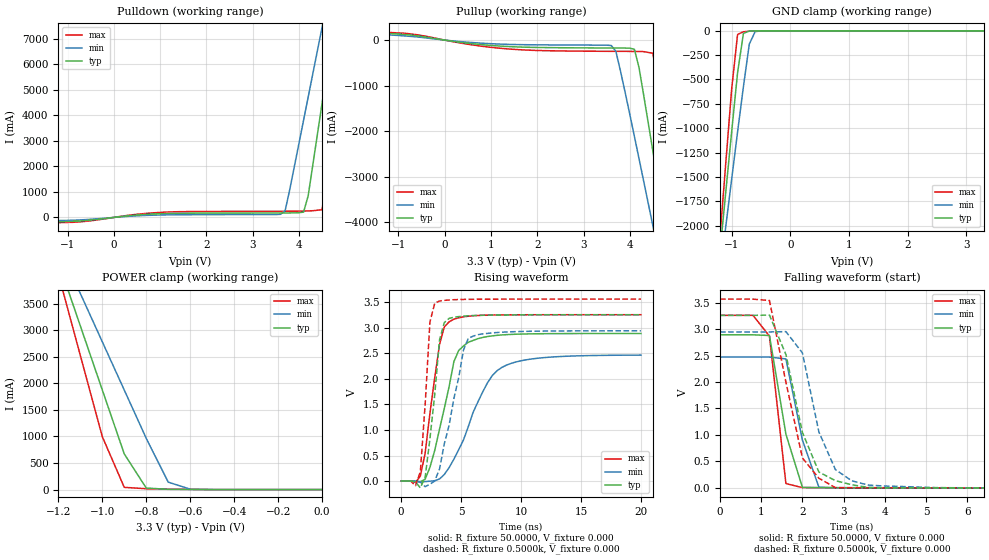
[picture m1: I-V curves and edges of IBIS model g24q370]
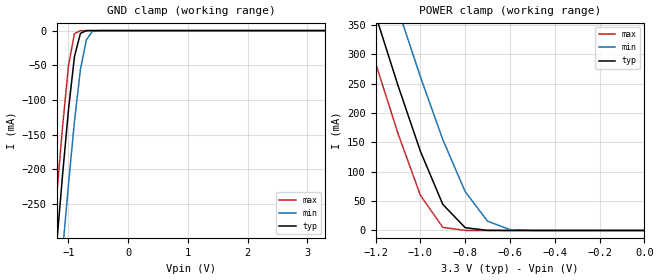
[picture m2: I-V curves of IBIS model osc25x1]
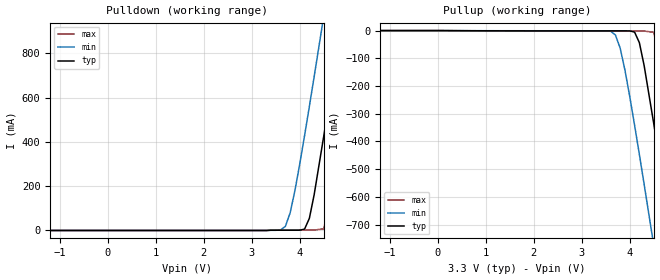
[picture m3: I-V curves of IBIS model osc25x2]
|   National Semiconductor Corporation
|   Interface Products Group
|   IBIS Model of DP83849
|   80L LQFP Package
[IBIS Ver]   4.2
[Comment char]  |_char
[File name]   dp83849.ibs
[File Rev]   1.1
[Date]   09/07/2010
[Source]   File originated at National Semiconductor Corporation.
   Interface Group/Analog Division. All models created with
   Spectre s2ibis simulations by Sida Zhang.
   Originally Created on 8/24/2005 by Sida Zhang, modified
   on 9/07/2010 by Peggy Alavi
[Notes]
   Rev 0.1 The pins TPTDP, TPTDM, TPRDP, and TPRDM are
   high-speed analog I/O pins. Models of these pins are
   not available due to the IBIS modeling limitations
   and design complexity.
   Rev 1.1 removes model selector. Model selector included a
   production test mode which is not available in the final
   product.
Begin IBIS Parser Results
| Do NOT edit this section manually!
Checking ...\dp83849.ibs for IBIS 4.2 Compatibility...
WARNING - Model osc25x1: POWER Clamp : Typical value never becomes zero
WARNING - Model osc25x1: POWER Clamp : Minimum value never becomes zero
WARNING - Model osc25x1: POWER Clamp : Maximum value never becomes zero
Errors  : 0
Warnings: 3
File Passed
| End IBIS Parser Results
[Disclaimer]
(C) Copyright National Semiconductor Corporation 2010
   All rights reserved
   National Semiconductor Corporation hereby grants
the user of this IBIS model a non-exclusive, nontransferable
license to use this IBIS model under the following terms.
Before using this IBIS model, the user should read this
license.  If the user does not accept these terms,  the
IBIS model should be returned to National within 30 days.
   The user is granted this license only to use the
IBIS model and is not granted rights to sell, load, rent,
lease or license the IBIS model in whole or in part, or in
modified form to anyone other than user. User may modify
the IBIS model to suit its specific applications but rights
to derivative works and such modifications shall belong to
National.
   This IBIS model is provided on an "AS IS" basis and
National makes absolutely no warranty with respect to the
information contained herein.NATIONAL DISCLAIMS AND CUSTOMER
WAIVES ALL WARRANTIES, EXPRESS OR IMPLIED, INCLUDING
WARRANTIES OF MERCHANTABILITY OR FITNESS FOR A PARTICULAR
PURPOSE. The entire risk as to quality and performance is
with the Customer. ACCORDINGLY, IN NO EVENT SHALL THE
COMPANY BE LIABLE FOR ANY DAMAGES, WHETHER IN CONTRACT OR
TORT,INCLUDING ANY LOST PROFITS OR OTHER INCIDENTAL,
CONSEQUENTIAL, EXEMPLARY, OR PUNITIVE DAMAGES ARISING OUT
OF THE USE OR APPLICATION OF THE IBIS model provided in
this package.Further, National reserves the right to make
changes without notice to any product herein to improve
reliability, function, or design. National does not convey
any license under patent rights or any other intellectual
property rights, including those of third parties.
   National is not obligated to provide maintenance or support
for the licensed IBIS model.
[Copyright]   Copyright 2010, National Semiconductor, All Rights Reserved
[Component]   DP83849
[Manufacturer]  National Semiconductor Corporation
[Package]
|   typ   min   max
R_pkg   0.171   0.153   0.189
L_pkg   5.515nH   4.604nH   6.091nH
C_pkg   0.126pF   0.090p   0.273p
[Pin]   signal_name   model_name   R_pin   L_pin   C_pin
1   CRS_A   g24q370   0.18332   5.99n   0.273p
2   RX_ER_A   g24q370   0.1772   5.642n   0.124p
3   COL_A   g24q370   0.17474   5.41n   0.105p
4   RXD0_A   g24q370   0.17112   5.202n   0.097p
5   RXD1_A   g24q370   0.16808   5.036n   0.092p
6   COREGND1   GND   0.1654   4.894n   0.09p
7   PFBIN1   NC   0.16363   4.792n   0.09p
8   RXD2_A   g24q370   0.16189   4.711n   0.093p
9   RXD3_A   g24q370   0.16103   4.653n   0.102p
10   IOGND1   GND   0.15937   4.604n   0.183p
11   IOVDD1   POWER   0.15311   4.633n   0.184p
12   TX_CLK_A   g24q370   0.16419   4.867n   0.103p
13   TX_EN_A   g24q370   0.17125   4.867n   0.095p
14   TXD0_A   g24q370   0.17056   4.854n   0.092p
15   TXD1_A   g24q370   0.17201   4.92n   0.094p
16   TXD2_A   g24q370   0.17334   4.989n   0.095p
17   TXD3_A   g24q370   0.17521   5.099n   0.1p
18   PWRDOWN_INT_A   g24q370   0.17779   5.236n   0.105p
19   LED_LINK_A   g24q370   0.18792   5.842n   0.124p
20   LED_SPEED_A   g24q370   0.1893   6.091n   0.271p
21   LED_ACT/COL_A   g24q370   0.18332   5.99n   0.273p
22   ANAGND1   GND   0.1772   5.642n   0.124p
23   TPRDM_A   NC   0.17474   5.41n   0.105p
24   TPRDP_A   NC   0.17112   5.202n   0.097p
25   CDGND1   GND   0.16808   5.036n   0.092p
26   TPTDM_A   NC   0.1654   4.894n   0.09p
27   TPTDP_A   NC   0.16363   4.792n   0.09p
28   PFBIN2   NC   0.16189   4.711n   0.093p
29   ANAGND2   GND   0.16103   4.653n   0.102p
30   ANA33VDD   POWER   0.15937   4.604n   0.183p
31   PFBOUT   NC   0.15311   4.633n   0.184p
32   RBIAS   NC   0.16419   4.867n   0.103p
33   ANAGND3   GND   0.17125   4.867n   0.095p
34   PFBIN3   NC   0.17056   4.854n   0.092p
35   TPTDP_B   NC   0.17201   4.92n   0.094p
36   TPTDM_B   NC   0.17334   4.989n   0.095p
37   CDGND2   GND   0.17521   5.099n   0.1p
38   TPRDP_B   NC   0.17779   5.236n   0.105p
39   TPRDM_B   NC   0.18792   5.842n   0.124p
40   ANAGND4   GND   0.1893   6.091n   0.271p
41   LED_ACT/COL_B   g24q370   0.18332   5.99n   0.273p
42   LED_SPEED_B   g24q370   0.1772   5.642n   0.124p
43   LED_LINK_B   g24q370   0.17474   5.41n   0.105p
44   PWRDOWN_INT_B   g24q370   0.17112   5.202n   0.097p
45   TXD3_B   g24q370   0.16808   5.036n   0.092p
46   TXD2_B   g24q370   0.1654   4.894n   0.09p
47   TXD1_B   g24q370   0.16363   4.792n   0.09p
48   TXD0_B   g24q370   0.16189   4.711n   0.093p
49   TX_EN_B   g24q370   0.16103   4.653n   0.102p
50   TX_CLK_B   g24q370   0.15937   4.604n   0.183p
51   IOVDD2   POWER   0.15311   4.633n   0.184p
52   IOGND2   GND   0.16419   4.867n   0.103p
53   RXD3_B   g24q370   0.17125   4.867n   0.095p
54   PFBIN4   NC   0.17056   4.854n   0.092p
55   COREGND2   GND   0.17201   4.92n   0.094p
56   RXD2_B   g24q370   0.17334   4.989n   0.095p
57   RXD1_B   g24q370   0.17521   5.099n   0.1p
58   RXD0_B   g24q370   0.17779   5.236n   0.105p
59   COL_B   g24q370   0.18792   5.842n   0.124p
60   RX_ER_B   g24q370   0.1893   6.091n   0.271p
61   CRS_B   g24q370   0.18332   5.99n   0.273p
62   RX_DV_B   g24q370   0.1772   5.642n   0.124p
63   RX_CLK_B   g24q370   0.17474   5.41n   0.105p
64   IOGND3   GND   0.17112   5.202n   0.097p
65   IOVDD3   POWER   0.16808   5.036n   0.092p
66   MDIO   g24q370   0.1654   4.894n   0.09p
67   MDC   g24q370   0.16363   4.792n   0.09p
68   CLK2MAC   g24q370   0.16189   4.711n   0.093p
69   X2   osc25x2   0.16103   4.653n   0.102p
70   X1   osc25x1   0.15937   4.604n   0.183p
71   RESET_N   g24q370   0.15311   4.633n   0.184p
72   TCK   g24q370   0.16419   4.867n   0.103p
73   TDO   g24q370   0.17125   4.867n   0.095p
74   TMS   g24q370   0.17056   4.854n   0.092p
75   TRST_N   g24q370   0.17201   4.92n   0.094p
76   TDI   g24q370   0.17334   4.989n   0.095p
77   IOGND4   GND   0.17521   5.099n   0.1p
78   IOVDD4   POWER   0.17779   5.236n   0.105p
79   RX_CLK_A   g24q370   0.18792   5.842n   0.124p
80   RX_DV_A   g24q370   0.1893   6.091n   0.271p
[Diff_pin]   inv_pin   vdiff   tdelay_typ   tdelay_min   tdelay_max
| The '+' pin is Diff_pin and the '-' pin is the inv_pin
24   23   0.100   0 0 0
27   26   0.100   0 0 0
35   36   0.100   0 0 0
38   39   0.100   0 0 0
| Models and submodels in the file (3): g24q370 (I/O), osc25x1 (Input), osc25x2 (Output)
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|   Model g24q370
[Model]   g24q370
Model_type   I/O
Polarity   Non-Inverting
Enable   Active-High
Vinl = 0.8000V
Vinh = 2.0000V
Vmeas = 1.5000V
C_comp   1.0640pF   1.0620pF   1.0670pF
[Temperature Range]   25.0000   0.1250k   -40.0000
[Voltage Range]   3.3000V   3.0000V   3.6000V
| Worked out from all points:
|   slope of the pulldown table from 0 to 0.495 V, typ, clamps not added: 5.31 ohm
|   slope of the pullup table from 0 to 0.495 V, typ, clamps not added: 7.25 ohm
|   GND clamp passes 1 mA (typ) near -0.64 V on its own axis
|   POWER clamp passes 1 mA (typ) near -0.54 V on its own axis
|   rising waveform, R_fixture 50.0000, V_fixture 0.000: 20-80 % time 1.6ns typ, 2.8ns min, 1.1ns max; typ from 0 V to 2.89 V
|   rising waveform, R_fixture 0.5000k, V_fixture 0.000: 20-80 % time 833ps typ, 1.56ns min, 573ps max; typ from 0 V to 3.26 V
|   falling waveform, R_fixture 50.0000, V_fixture 0.000: 20-80 % time 452ps typ, 464ps min, 281ps max; typ from 2.89 V to 0 V
|   falling waveform, R_fixture 0.5000k, V_fixture 0.000: 20-80 % time 659ps typ, 611ps min, 580ps max; typ from 3.26 V to 0 V
[Pulldown]
| voltage   I(typ)   I(min)   I(max)
-3.3V     -160.5mA   -118.3mA   -200.7mA
-900mV    -153.7mA   -111mA     -192.4mA
1.1V      151.8mA    98.11mA    206.2mA
3.6V      174.1mA    121.6mA    241.2mA
3.7V      174.7mA    254.1mA    242mA
4.1V      208.2mA    3.809A     248.7mA
4.2V      852.2mA    4.721A     254.3mA
4.5V      4.477A     7.457A     302mA
4.7V      6.898A     9.283A     2.796A
4.9V      9.321A     11.11A     5.87A
5.1V      11.75A     12.94A     8.947A
6.6V      30.05A     26.73A     32.17A
[Pullup]
| voltage   I(typ)   I(min)   I(max)
-3.3V     188.1mA    165.2mA    206.9mA
-900mV    123.6mA    93.95mA    153.1mA
1.3V      -138.1mA   -91.87mA   -188.7mA
3.6V      -174.3mA   -119.7mA   -247.2mA
3.7V      -174.6mA   -248.3mA   -247.7mA
4.1V      -202.3mA   -2.118A    -249.5mA
4.2V      -607mA     -2.608A    -250.6mA
4.5V      -2.447A    -4.087A    -288.9mA
4.7V      -3.699A    -5.076A    -1.602A
4.9V      -4.956A    -6.068A    -3.14A
5.1V      -6.215A    -7.061A    -4.687A
6.6V      -15.68A    -14.52A    -16.34A
[GND_clamp]
| voltage   I(typ)   I(min)   I(max)
-3.3V     -15.47A    -12.9A     -18.37A
-1.2V     -2.269A    -2.494A    -2.116A
-1.1V     -1.647A    -2.005A    -1.349A
-1V       -1.031A    -1.519A    -592.6mA
-900mV    -430.7mA   -1.039A    -37.49mA
-800mV    -26.32mA   -572.9mA   -9.444mA
-700mV    -1.926mA   -136.4mA   -3.598mA
-600mV    -247.7uA   -8.119mA   -648.8uA
-400mV    -1.571uA   -27.47uA   -1.62uA
3.3V      22.02pA    3.648uA    15.2pA
[POWER_clamp]
| voltage   I(typ)   I(min)   I(max)
-3.3V     29.64A     23.74A     36.19A
-1.2V     4.29A      4.604A     4.058A
-1.1V     3.083A     3.693A     2.528A
-1V       1.877A     2.784A     997.8mA
-900mV    671.8mA    1.874A     42.61mA
-800mV    29.37mA    964.9mA    16.3mA
-700mV    5.409mA    140.5mA    9.688mA
-600mV    1.864mA    8.479mA    4.466mA
0V        22.02pA    589.3pA    18.15pA
[Ramp]
| variable   typ   min   max
dV/dt_r   1.7348/1.6680n   1.4811/3.0471n   1.9560/1.1060n
dV/dt_f   1.8068/1.8411n   1.5594/3.2593n   2.0132/1.2189n
R_load = 50.0000
[Rising Waveform]
R_fixture = 50.0000
V_fixture = 0.000
V_fixture_min = 0.000
V_fixture_max = 0.000
| time   V(typ)   V(min)   V(max)
0s        121pV      6.465nV    36.64pV
1.6ns     -12.04mV   -15.26mV   96.9mV
2ns       34.22mV    -11.2mV    543.1mV
2.4ns     268mV      -3.569mV   1.326V
3.2ns     1.016V     39.7mV     2.674V
4ns       1.85V      262mV      3.12V
4.8ns     2.559V     613.5mV    3.2V
7.2ns     2.832V     1.925V     3.252V
8.4ns     2.864V     2.227V     3.257V
20ns      2.891V     2.468V     3.26V
[Rising Waveform]
R_fixture = 0.5000k
V_fixture = 0.000
V_fixture_min = 0.000
V_fixture_max = 0.000
| time   V(typ)   V(min)   V(max)
0s        130pV      7.171nV    38.79pV
1.2ns     -20.26mV   28.89uV    -92.41mV
1.6ns     -134.2mV   -21.16mV   180.7mV
2ns       72.06mV    -111.1mV   1.492V
2.4ns     825.8mV    -63.59mV   3.114V
2.8ns     1.692V     781.9uV    3.485V
3.2ns     2.765V     233.9mV    3.529V
3.6ns     3.107V     729.7mV    3.542V
5.6ns     3.239V     2.796V     3.562V
20ns      3.259V     2.945V     3.566V
[Falling Waveform]
R_fixture = 50.0000
V_fixture = 0.000
V_fixture_min = 0.000
V_fixture_max = 0.000
| time   V(typ)   V(min)   V(max)
0s        2.891V     2.471V     3.26V
800ps     2.891V     2.471V     3.26V
1.2ns     2.878V     2.471V     2.867V
1.6ns     1.014V     2.436V     81.31mV
2ns       8.918mV    903.1mV    5.147mV
2.4ns     3.412mV    11.78mV    4.297mV
20ns      2.471uV    23.79uV    19.15uV
[Falling Waveform]
R_fixture = 0.5000k
V_fixture = 0.000
V_fixture_min = 0.000
V_fixture_max = 0.000
| time   V(typ)   V(min)   V(max)
0s        3.259V     2.945V     3.566V
1.2ns     3.265V     2.946V     3.539V
1.6ns     2.519V     2.952V     1.996V
2ns       1.048V     2.55V      564.1mV
2.4ns     298.8mV    1.056V     181.6mV
2.8ns     136.3mV    345.2mV    4.978mV
3.2ns     58.01mV    132.1mV    1.436mV
3.6ns     8.285mV    52.25mV    931.6uV
5.2ns     739.4uV    5.88mV     479.6uV
20ns      3.35uV     19.65uV    13.62uV
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|   Model osc25x1
[Model]   osc25x1
Model_type   Input
Polarity   Inverting
Enable   Active-High
Vinl = 0.8000V
Vinh = 2.0000V
C_comp   1.0000pF   1.0000pF   1.0000pF
[Temperature Range]   25.0000   0.1250k   -40.0000
[Voltage Range]   3.3000V   3.0000V   3.6000V
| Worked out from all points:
|   GND clamp passes 1 mA (typ) near -0.72 V on its own axis
|   POWER clamp passes 1 mA (typ) near -0.72 V on its own axis
[GND_clamp]
| voltage   I(typ)   I(min)   I(max)
-3.3V     -2.622A    -2.694A    -2.579A
-1.3V     -414.8mA   -523mA     -346.4mA
-1.2V     -310.3mA   -419.8mA   -240.9mA
-1.1V     -208.9mA   -318.8mA   -139.7mA
-1V       -114.1mA   -221.5mA   -50.66mA
-900mV    -37.58mA   -131mA     -4.515mA
-800mV    -4.019mA   -56.03mA   -47.48uA
-700mV    -108.1uA   -13.33mA   -2.355uA
-600mV    -3.685uA   -1.282mA   -1.753uA
-400mV    -1.001uA   -4.899uA   -1.167uA
3.3V      8.25uA     7.477uA    9.629uA
[POWER_clamp]
| voltage   I(typ)   I(min)   I(max)
-3.3V     3.1A       3.186A     3.05A
-1.3V     490.5mA    618.5mA    409.7mA
-1.2V     366.9mA    496.4mA    284.9mA
-1.1V     247mA      377mA      165.2mA
-1V       135mA      261.9mA    59.9mA
-900mV    44.44mA    154.8mA    5.346mA
-800mV    4.759mA    66.25mA    66.21uA
-700mV    135.7uA    15.76mA    12.92uA
-600mV    12.33uA    1.522mA    12.26uA
-500mV    9.553uA    95.08uA    11.96uA
0V        8.25uA     6.563uA    10.5uA
|   Model osc25x2
[Model]   osc25x2
Model_type   Output
Polarity   Inverting
Enable   Active-High
Vmeas = 1.5000V
C_comp   1.0000pF   1.0000pF   1.0000pF
[Temperature Range]   25.0000   0.1250k   -40.0000
[Voltage Range]   3.3000V   3.0000V   3.6000V
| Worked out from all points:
|   slope of the pullup table from 0 to 0.495 V, typ, clamps not added: 1.19 kohm
[Pulldown]
| voltage   I(typ)   I(min)   I(max)
-3.3V     0A         0A         0A
3.6V      1.099mA    2.318mA    1.555mA
3.7V      1.103mA    18.37mA    1.56mA
3.8V      1.11mA     80.08mA    1.567mA
4.1V      6.217mA    428mA      1.603mA
4.2V      54.57mA    559.8mA    1.639mA
4.5V      425.9mA    967.9mA    7.417mA
4.7V      707.9mA    1.245A     200.5mA
4.9V      996mA      1.525A     486.1mA
5.1V      1.287A     1.806A     783.4mA
5.3V      1.58A      2.089A     1.085A
6.6V      3.503A     3.939A     3.076A
[Pullup]
| voltage   I(typ)   I(min)   I(max)
-3.3V     0A         0A         0A
3.6V      -1.081mA   -2.06mA    -1.527mA
3.7V      -1.083mA   -15.55mA   -1.53mA
3.8V      -1.086mA   -63.14mA   -1.534mA
4.1V      -5.367mA   -340.7mA   -1.543mA
4.2V      -43.48mA   -446.6mA   -1.551mA
4.5V      -335.7mA   -775mA     -6.395mA
4.7V      -559.6mA   -998.5mA   -156mA
4.9V      -788.6mA   -1.224A    -379.2mA
5.1V      -1.02A     -1.451A    -612.3mA
5.3V      -1.253A    -1.678A    -849mA
6.6V      -2.784A    -3.17A     -2.413A
[Ramp]
| variable   typ   min   max
dV/dt_r   1.7737/0.4988n   1.5328/0.7567n   1.9870/0.3615n
dV/dt_f   1.8364/0.4766n   1.5967/0.7630n   2.0404/0.3438n
R_load = 10.0000k
